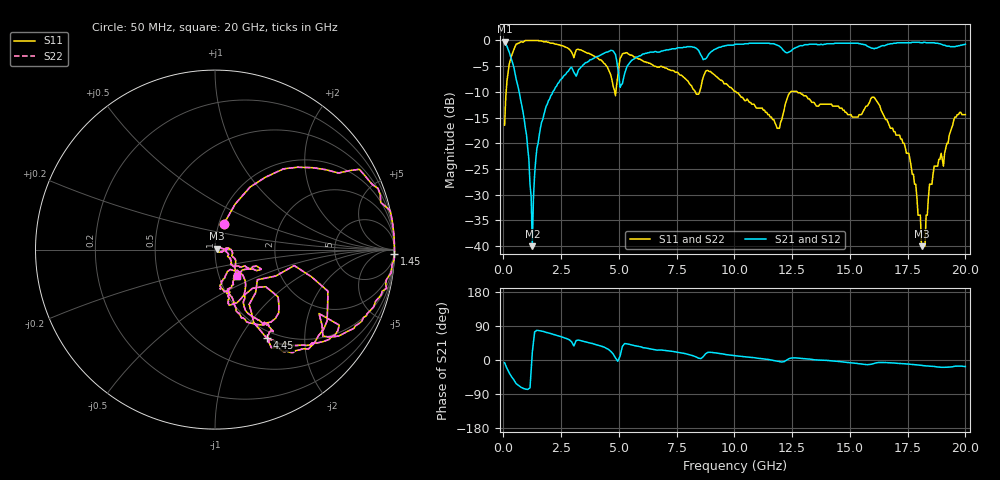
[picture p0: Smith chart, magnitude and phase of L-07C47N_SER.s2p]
#	mhz	s	ma	r	50
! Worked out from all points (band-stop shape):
!   400 points, 50 MHz to 20 GHz, reference 50 ohm
!   highest |S21| = -0.26 dB at 50 MHz (marker M1); lowest = -40.0 dB at 1.25 GHz (marker M2)
!   |S21| within 3 dB of the highest: 5.742 GHz to 8.604 GHz (2.862 GHz wide, 39.9 % of centre); 8.811 GHz to end of sweep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
!   lowest |S11| = -40.0 dB at 18.1 GHz (marker M3), VSWR 1.02, Z = 50.9 + j0.473 ohm
!   |S11| at or under -10 dB: 8.309 GHz to 8.491 GHz (181.6 MHz wide, 2.16 % of centre); 10.07 GHz to 12.43 GHz (2.363 GHz wide, 21 % of centre); 12.72 GHz to end of sweep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
!   |S22| runs from -40.0 to 0.0 dB; largest |S21 - S12| = 0
!   S11 on the Smith chart (normalised r, x): 50 MHz: 1.06, +0.31; 1.45 GHz: 0, -76; 4.45 GHz: 0.90, -1.32; 20 GHz: 1.22, -0.37
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50  0.15 71.2  0.97 -7.1  0.97 -7.1  0.15 71.2
250  0.59 49.7  0.77 -34.0  0.77 -34.0  0.59 49.7
1000  1 10.9  0.12 -77.2  0.12 -77.2  1 10.9
1200  1 5.1  0.03 -26.6  0.03 -26.6  1 5.1
1250  1 4.0  0.01 20.4  0.01 20.4  1 4.0
1300  1 2.2  0.03 47.3  0.03 47.3  1 2.2
1450  1 -1.5  0.09 78.3  0.09 78.3  1 -1.5
2150  0.94 -19.8  0.32 68.0  0.32 68.0  0.94 -19.8
3400  0.8 -39.3  0.56 50.3  0.56 50.3  0.8 -39.3
4450  0.57 -59.5  0.77 31.2  0.77 31.2  0.57 -59.5
4950  0.45 -11.4  0.54 -3.4  0.54 -3.4  0.45 -11.4
5350  0.76 -46.7  0.56 42.6  0.56 42.6  0.76 -46.7
6700  0.55 -55.6  0.77 26.2  0.77 26.2  0.55 -55.6
10050  0.32 -70.7  0.92 11.2  0.92 11.2  0.32 -70.7
11850  0.14 -60.4  0.9 -3.0  0.9 -3.0  0.14 -60.4
12450  0.32 -67.4  0.79 5.1  0.79 5.1  0.32 -67.4
13350  0.25 -70.6  0.92 1.5  0.92 1.5  0.25 -70.6
16700  0.15 -37.7  0.92 -7.3  0.92 -7.3  0.15 -37.7
17550  0.08 -18.9  0.95 -10.8  0.95 -10.8  0.08 -18.9
18100  0.01 27.7  0.95 -14.2  0.95 -14.2  0.01 27.7
18650  0.06 5.0  0.95 -17.1  0.95 -17.1  0.06 5.0
20000  0.19 -49.8  0.92 -17.3  0.92 -17.3  0.19 -49.8
